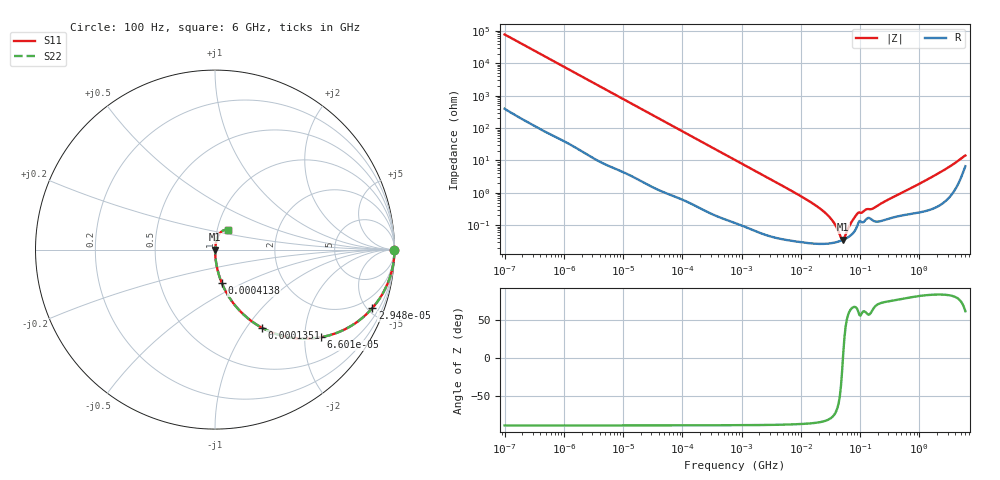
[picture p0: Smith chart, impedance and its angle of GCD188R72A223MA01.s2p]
!Murata Part Number: GCD188R72A223MA01
!These Parameters are Measured in Series Mode Connection
!Data Generated on Mar 13, 2026
!  o--ll--o
!Port1  Port2
!  o------o
!Operation Temp=25[degC], DC Bias Voltage=0[V]
!Freq. Start=100[Hz] Stop=6[GHz] 401[Steps]
# Hz S RI R 50
!Freq.(Hz) S11(Real) S11(Imag) S21(Real) S21(Imag) S12(Real) S12(Imag) S22(Real) S22(Imag)
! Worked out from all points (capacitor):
!   401 points, 100 Hz to 6 GHz, reference 50 ohm
!   read as one part in series: C = 20.4 nF near 109 Hz
!   lowest |Z| = 35.6 mohm at 52.11 MHz (marker M1)
!   series resonance near 51.45 MHz, so ESL is about 470 pH
!   S11 on the Smith chart (normalised r, x): 100 Hz: open; 29.48 kHz: 1.03, -5.37; 66 kHz: 1.02, -2.40; 135.1 kHz: 1.01, -1.18; 413.8 kHz: 1.00, -0.39; 6 GHz: 1.13, +0.25
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100  1 -0.00129  8.2e-06 0.00129  8.2e-06 0.00129  1 -0.00129
2008  0.9992 -0.0256  0.000779 0.0256  0.000779 0.0256  0.9992 -0.0256
9204  0.9859 -0.1151  0.0141 0.1151  0.0141 0.1151  0.9859 -0.1151
29482  0.8767 -0.3258  0.1233 0.3258  0.1233 0.3258  0.8767 -0.3258
40335  0.7927 -0.4023  0.2073 0.4023  0.2073 0.4023  0.7927 -0.4023
66005  0.5905 -0.4883  0.4095 0.4883  0.4095 0.4883  0.5905 -0.4883
135116  0.2596 -0.4344  0.7404 0.4344  0.7404 0.4344  0.2596 -0.4344
221108  0.1175 -0.3178  0.8825 0.3178  0.8825 0.3178  0.1175 -0.3178
413847  0.0377 -0.1859  0.9623 0.1859  0.9623 0.1859  0.0377 -0.1859
774597  0.0118 -0.1024  0.9882 0.1024  0.9882 0.1024  0.0118 -0.1024
1.555665e7  0.000294 -0.00479  0.9997 0.00479  0.9997 0.00479  0.000294 -0.00479
3.045065e7  0.000275 -0.00176  0.9997 0.00176  0.9997 0.00176  0.000275 -0.00176
3.80911e7  0.000293 -0.000983  0.9997 0.000983  0.9997 0.000983  0.000293 -0.000983
4.764863e7  0.000331 -0.000249  0.9997 0.000249  0.9997 0.000249  0.000331 -0.000249
5.211241e7  0.000353 4.21e-05  0.9996 -4.21e-05  0.9996 -4.21e-05  0.000353 4.21e-05
7.129496e7  0.000504 0.00111  0.9995 -0.00111  0.9995 -0.00111  0.000504 0.00111
8.918374e7  0.000927 0.00202  0.9991 -0.00202  0.9991 -0.00202  0.000927 0.00202
1.275994e8  0.00154 0.00265  0.9985 -0.00265  0.9985 -0.00265  0.00154 0.00265
1.669249e8  0.00138 0.00298  0.9986 -0.00298  0.9986 -0.00298  0.00138 0.00298
3.124326e8  0.00164 0.0062  0.9984 -0.0062  0.9984 -0.0062  0.00164 0.0062
1.637704e9  0.00406 0.0305  0.9959 -0.0305  0.9959 -0.0305  0.00406 0.0305
6e9  0.0748 0.1087  0.9252 -0.1087  0.9252 -0.1087  0.0748 0.1087
